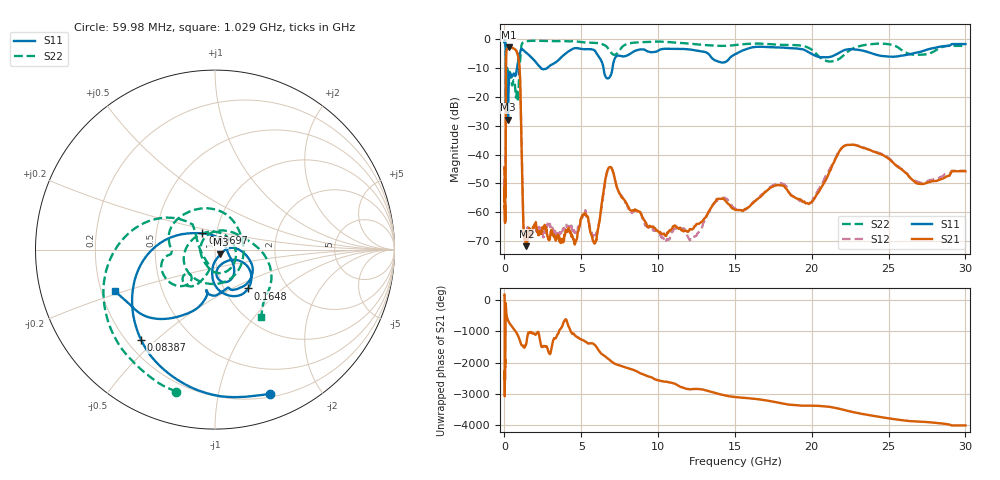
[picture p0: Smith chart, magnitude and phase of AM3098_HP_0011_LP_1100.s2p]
! Date/Time: Thu, Feb 28, 2019 8:34 AM
! Network Analyzer: Agilent Technologies E8364B Rev: A.07.50.67
! Sweep from 0.010 to 30.000 GHz, 1601 Points, Sweep Type: LOG
! Power Supply: 5.023 V, 0.002 A
# Hz S DB R 50
!freq MagS11 AngS11 MagS21 AngS21 MagS12 AngS12 MagS22 AngS22
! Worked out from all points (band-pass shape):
!   1601 points, 10 MHz to 30 GHz, reference 50 ohm
!   highest |S21| = -2.80 dB at 269.1 MHz (marker M1); lowest = -71.8 dB at 1.432 GHz (marker M2)
!   |S21| within 3 dB of the highest: 108.5 MHz to 888.3 MHz (779.7 MHz wide, 156 % of centre)
!   lowest |S11| = -27.9 dB at 233.9 MHz (marker M3), VSWR 1.08, Z = 53 - j2.88 ohm
!   |S11| at or under -10 dB: 93.02 MHz to 811.5 MHz (718.5 MHz wide, 159 % of centre); 2.376 GHz to 2.769 GHz (393 MHz wide, 15.3 % of centre); 6.448 GHz to 7.033 GHz (585.1 MHz wide, 8.68 % of centre)
!   |S22| runs from -22.5 to -0.5 dB; largest |S21 - S12| = 0.011
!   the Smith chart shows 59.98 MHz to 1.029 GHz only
!   S11 on the Smith chart (normalised r, x): 59.98 MHz: 0.23, -1.43; 83.87 MHz: 0.26, -0.45; 96.97 MHz: 0.86, +0.16; 164.8 MHz: 1.29, -0.61; 1.029 GHz: 0.26, -0.19
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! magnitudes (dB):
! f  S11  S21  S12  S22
! 10 MHz  -0.4  -45.0  -44.4  -0.6
! 38.04 MHz  -0.5  -59.0  -60.3  -1.0
! 59.98 MHz  -1.3  -51.6  -52.1  -1.7
! 83.87 MHz  -3.7  -35.4  -35.3  -4.2
! 96.97 MHz  -18.8  -11.2  -11.2  -21.5
! 144.7 MHz  -15.5  -3.5  -3.5  -13.0
! 164.8 MHz  -10.9  -3.4  -3.3  -10.3
! 233.9 MHz  -27.9  -2.9  -2.9  -12.1
! 269.1 MHz  -16.9  -2.8  -2.8  -12.3
! 550.5 MHz  -12.3  -3.1  -3.0  -14.9
! 885.5 MHz  -7.7  -5.7  -5.7  -21.7
! 1.029 GHz  -4.4  -15.7  -15.7  -6.8
! 1.238 GHz  -3.8  -65.2  -64.7  -1.0
! 1.432 GHz  -4.6  -71.8  -68.3  -0.6
! 2.084 GHz  -8.2  -65.4  -66.4  -0.5
! 5.841 GHz  -3.7  -70.8  -67.3  -1.2
! 6.855 GHz  -13.1  -44.3  -44.3  -3.9
! 7.926 GHz  -5.7  -56.8  -56.9  -1.7
! 12.31 GHz  -3.7  -65.6  -69.2  -1.6
! 19.8 GHz  -4.5  -57.2  -56.8  -3.0
! 22.56 GHz  -3.4  -36.6  -36.6  -3.5
! 30 GHz  -1.6  -45.8  -45.6  -2.3
